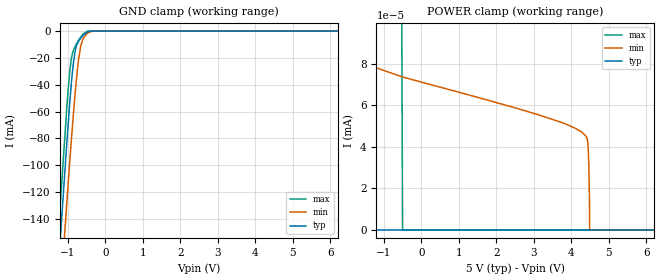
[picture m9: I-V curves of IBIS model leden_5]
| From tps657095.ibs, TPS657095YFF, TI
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|   leden_5 Model
[Model]   leden_5
Model_type   Input
Vinl = 0.4
Vinh = 1.2
|   typ   min   max
|   (nom PVT)   (fast PVT)   (slow PVT)
C_comp   1.794e-12   1.720e-12   1.893e-12
| Where nom  PVT is Nominal Process, 5V, 27C
|   Fast PVT is Strong Process,  5.5V, -40C
|   Slow PVT is Weak Process,   4.5V, 125C
[Voltage Range]   5   4.5   5.5
|Junction Temperature
[Temperature Range]   27   125   -40
[Power Clamp Reference]   5   4.5   5.5
[GND Clamp Reference]   0   0   0
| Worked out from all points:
|   GND clamp passes 1 mA (typ) near -0.50 V on its own axis
|   POWER clamp passes 1 mA (typ) near -3.66 V on its own axis
[GND Clamp]
|   Voltage   I(typ)   I(min)   I(max)
-5V       -1.942A    -1.92A     -1.969A
-1.252V   -175.4mA   -218.1mA   -150.5mA
-1.19V    -149.1mA   -192.6mA   -123.3mA
-1.022V   -80.11mA   -124.6mA   -53.74mA
-957.5mV  -55.78mA   -99.65mA   -31.77mA
-915mV    -41.11mA   -83.7mA    -21.6mA
-846.5mV  -21.94mA   -59.22mA   -13.83mA
-750mV    -9.403mA   -29.37mA   -8.438mA
-662mV    -5.381mA   -11.57mA   -4.525mA
-599mV    -3.279mA   -5.704mA   -2.309mA
-500mV    -962.3uA   -2.113mA   -348.9uA
10V       0A         0A         0A
[POWER Clamp]
|   Voltage   I(typ)   I(min)   I(max)
-5V       122.2mA    64.55mA    178.2mA
-3.525V   6.894uA    94.84nA    33.99mA
-3.389V   36.04nA    93.23nA    21.28mA
-3.273V   0A         91.96nA    11.05mA
-3.026V   0A         89.47nA    11.97uA
-500mV    0A         73.62nA    0A
4.297V    0A         46.88nA    0A
4.445V    0A         40.96nA    0A
4.473V    0A         27.09nA    0A
4.486V    0A         13.12nA    0A
4.49V     0A         0A         0A
10V       0A         0A         0A
